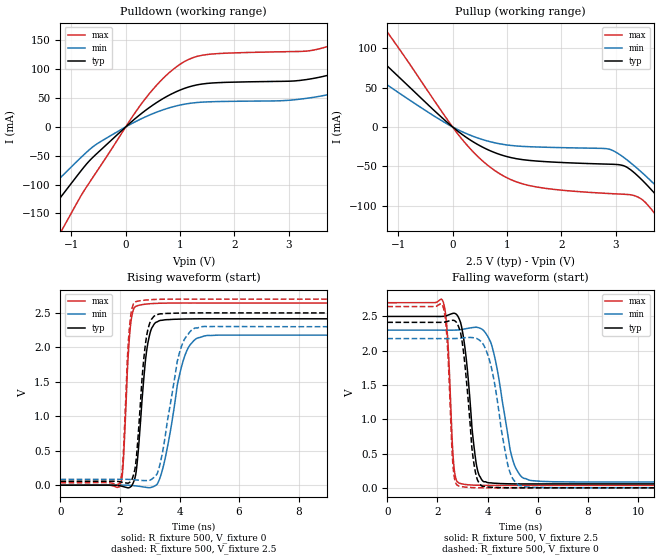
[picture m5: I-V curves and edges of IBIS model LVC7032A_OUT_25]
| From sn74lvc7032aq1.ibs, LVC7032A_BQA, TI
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[Model]   LVC7032A_OUT_25
Model_type  Output
Vref =   0
Rref =   500
Cref =   30p
Vmeas =   1.25
| variable   typ   min   max
C_comp   6.41pF   4.40pF   9.02pF
| C_pullup   5.80pF   4.43pF   6.82pF
| C_pulldown   7.02pF   4.40pF   9.02pF
[Temperature Range]   40   100   -40
| Ambient temperature   25   85   -40
[Voltage range]   2.5   2.3   2.7
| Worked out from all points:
|   slope of the pulldown table from 0 to 0.375 V, typ, clamps not added: 12.7 ohm
|   slope of the pullup table from 0 to 0.375 V, typ, clamps not added: 20 ohm
|   rising waveform, R_fixture 500, V_fixture 0: 20-80 % time 279ps typ, 541ps min, 178ps max; typ from 0 V to 2.41 V
|   falling waveform, R_fixture 500, V_fixture 2.5: 20-80 % time 369ps typ, 604ps min, 196ps max; typ from 2.5 V to 0.057 V
|   rising waveform, R_fixture 500, V_fixture 2.5: 20-80 % time 266ps typ, 509ps min, 170ps max; typ from 0.057 V to 2.5 V
|   falling waveform, R_fixture 500, V_fixture 0: 20-80 % time 350ps typ, 592ps min, 192ps max; typ from 2.41 V to 0 V
[Pulldown]
| LVC7032A_OUT_25
|   Voltage   I(typ)   I(min)   I(max)
-5.5V     -598.1mA   -479.8mA   -766.5mA
-2.12V    -233mA     -174.4mA   -327.1mA
-1.575V   -168.1mA   -123.2mA   -244.7mA
-1.15V    -116.2mA   -83.21mA   -174.9mA
-565mV    -49.19mA   -31.72mA   -81.94mA
365mV     28.75mA    17.58mA    49.46mA
1.32V     73.05mA    42.4mA     122.5mA
4V        96.78mA    61.72mA    149.2mA
4.6V      117.3mA    77.78mA    177.9mA
5.77V     171.8mA    120.4mA    253.2mA
7.055V    245.3mA    179.5mA    351.5mA
11V       504.9mA    394.6mA    686.5mA
[Pullup]
| LVC7032A_OUT_25
|   Voltage   I(typ)   I(min)   I(max)
-5.5V     363.4mA    279.9mA    508.8mA
-2.6V     169.4mA    122.6mA    251.6mA
-1.815V   117.7mA    83.03mA    179.1mA
-1.37V    88.47mA    61.37mA    136.9mA
170mV     -9.222mA   -5.867mA   -15.32mA
760mV     -32.2mA    -19.89mA   -54.58mA
2.905V    -47.35mA   -28.79mA   -84.65mA
3.45V     -65.04mA   -55.88mA   -90.57mA
3.92V     -100.7mA   -87.07mA   -129.3mA
4.19V     -123.8mA   -106.6mA   -157.6mA
4.495V    -151.4mA   -129.7mA   -191.8mA
11V       -830.2mA   -699.2mA   -1.022A
[Ramp]
| LVC7032A_OUT_25
| variable   typ   min   max
dV/dt_r   1.47/2.95E-10   1.33/5.87E-10   1.61/1.90E-10
dV/dt_f   1.49/4.03E-10   1.35/6.68E-10   1.63/2.09E-10
R_load = 500
[Rising Waveform]
| LVC7032A_OUT_25
R_fixture =   500
C_fixture =   0
L_fixture =   0
V_fixture =   0
V_fixture_min = 0
V_fixture_max = 0
|   Time   V(typ)   V(min)   V(max)
0s        177.7pV    3.876nV    17.91pV
1.995ns   -8.25mV    726.9uV    -10.63mV
2.105ns   -19.79mV   991.3uV    301.4mV
2.35ns    -25.73mV   -2.154mV   2.304V
2.635ns   608.5mV    -15.63mV   2.611V
3.075ns   2.287V     -28.4mV    2.636V
3.455ns   2.397V     271.3mV    2.642V
4.17ns    2.412V     1.87V      2.644V
4.84ns    2.415V     2.167V     2.644V
24.99ns   2.414V     2.176V     2.644V
[Falling Waveform]
| LVC7032A_OUT_25
R_fixture =   500
C_fixture =   0
L_fixture =   0
V_fixture =   2.5
V_fixture_min = 2.3
V_fixture_max = 2.7
|   Time   V(typ)   V(min)   V(max)
0s        2.5V       2.3V       2.7V
2.22ns    2.501V     2.3V       2.719V
2.405ns   2.517V     2.299V     2.184V
2.645ns   2.546V     2.3V       353.2mV
2.865ns   2.464V     2.304V     67mV
3.54ns    361.2mV    2.342V     37.74mV
3.855ns   87.67mV    2.286V     35.84mV
5.005ns   57.49mV    399.2mV    35.66mV
5.65ns    56.53mV    112.2mV    35.85mV
24.99ns   57.33mV    84.96mV    35.94mV
[Rising Waveform]
| LVC7032A_OUT_25
R_fixture =   500
C_fixture =   0
L_fixture =   0
V_fixture =   2.5
V_fixture_min = 2.3
V_fixture_max = 2.7
|   Time   V(typ)   V(min)   V(max)
0s        57.33mV    84.96mV    35.94mV
1.99ns    49.89mV    85.5mV     31.92mV
2.095ns   40.88mV    85.65mV    329mV
2.32ns    40.23mV    83.33mV    2.298V
2.555ns   423.9mV    75.22mV    2.667V
2.81ns    1.878V     66.86mV    2.684V
3.02ns    2.377V     75.96mV    2.692V
4.015ns   2.498V     1.947V     2.7V
4.53ns    2.5V       2.281V     2.7V
24.99ns   2.5V       2.3V       2.7V
[Falling Waveform]
| LVC7032A_OUT_25
R_fixture =   500
C_fixture =   0
L_fixture =   0
V_fixture =   0
V_fixture_min = 0
V_fixture_max = 0
|   Time   V(typ)   V(min)   V(max)
0s        2.414V     2.176V     2.644V
2.21ns    2.415V     2.176V     2.654V
2.385ns   2.426V     2.176V     2.138V
2.62ns    2.443V     2.177V     313.9mV
2.85ns    2.342V     2.18V      25.14mV
3.445ns   368.4mV    2.188V     2.282mV
3.79ns    22.16mV    2.114V     52.24uV
4.81ns    370.4uV    321.3mV    -211.3uV
5.275ns   -683.8uV   33.21mV    -86.56uV
24.99ns   12.59nV    -3.111nV   -7.211pV
